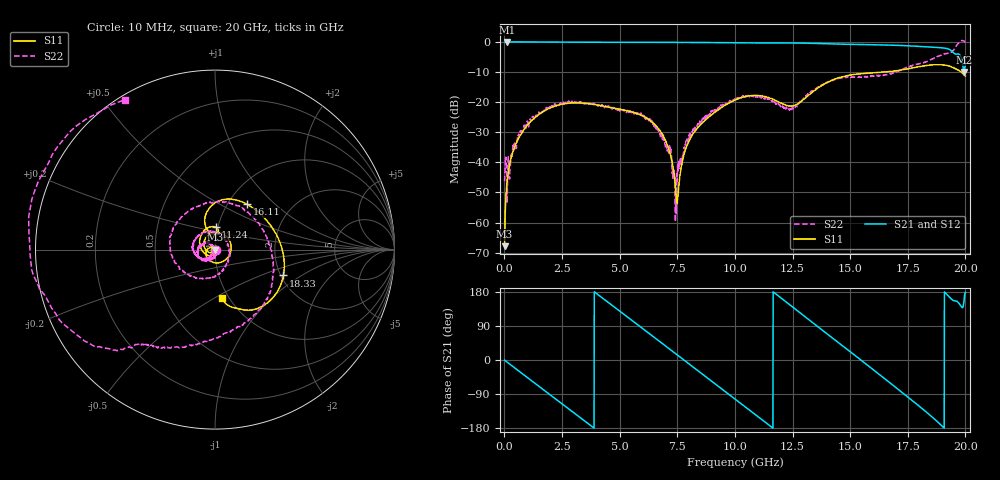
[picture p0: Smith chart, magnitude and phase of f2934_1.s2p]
!Keysight Technologies,M9372A,MY54321350,A.13.90.07
!Automatic Fixture Removal (AFR)
!Date: Wednesday, January 06, 2021, 09:20:31
!S2P File: Measurements: S11,S21,S12,S22:
# MHz S  RI  R 50
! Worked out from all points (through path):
!   2000 points, 10 MHz to 20 GHz, reference 50 ohm
!   highest |S21| = 0.03 dB at 110 MHz (marker M1); lowest = -9.9 dB at 19.94 GHz (marker M2)
!   group delay of S21, straight-line fit = 130 ps
!   lowest |S11| = -67.8 dB at 10 MHz (marker M3), VSWR 1.00, Z = 50 - j0.0401 ohm
!   |S11| at or under -10 dB: start of sweep to 16.5 GHz; 19.82 GHz to end of sweep
!   |S22| runs from -59.7 to 0.5 dB; largest |S21 - S12| = 1.4e-15
!   S11 on the Smith chart (normalised r, x): 10 MHz: 1.00, -0.00; 11.24 GHz: 0.98, +0.25; 16.11 GHz: 1.23, +0.68; 18.33 GHz: 2.07, -0.71; 20 GHz: 0.93, -0.54
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10  6.53e-05 -0.000401  1.001 -0.00816  1.001 -0.00816  0.00378 -0.00302
110  -0.00032 -0.00443  0.9996 -0.0893  0.9996 -0.0893  0.0053 0.000189
570  -0.0154 -0.0175  0.8976 -0.4467  0.8976 -0.4467  0.00109 -0.0249
1780  -0.0618 0.0397  0.1299 -0.9887  0.1299 -0.9887  -0.0467 -0.0594
3350  0.0657 0.0711  -0.8957 -0.4217  -0.8957 -0.4217  -0.1012 -0.0108
4270  0.0818 -0.0279  -0.9452 0.2919  -0.9452 0.2919  -0.0842 0.0183
5280  -0.00757 -0.0723  -0.436 0.8846  -0.436 0.8846  -0.0619 0.0304
6680  -0.0357 0.00734  0.6127 0.7702  0.6127 0.7702  -0.0207 0.0258
7500  0.00194 0.000737  0.9545 0.2282  0.9545 0.2282  -0.00469 -0.00127
8140  -0.00319 -0.0278  0.9399 -0.2749  0.9399 -0.2749  -0.0192 -0.0258
10010  -0.0801 0.0735  -0.222 -0.9425  -0.222 -0.9425  -0.1089 -0.0289
11240  0.00316 0.1255  -0.9081 -0.3201  -0.9081 -0.3201  -0.0798 0.0845
12220  0.00787 0.0885  -0.8581 0.4307  -0.8581 0.4307  0.0618 0.0509
13340  -0.0541 0.1344  -0.1658 0.9341  -0.1658 0.9341  -0.0095 -0.1539
14880  0.0313 0.275  0.8109 0.4234  0.8109 0.4234  -0.2372 0.1045
16110  0.1785 0.2521  0.7725 -0.4574  0.7725 -0.4574  0.1221 0.246
16670  0.2495 0.2015  0.4772 -0.7471  0.4772 -0.7471  0.2741 0.102
18330  0.3812 -0.1437  -0.6212 -0.5458  -0.6212 -0.5458  0.0471 -0.4688
19580  0.1361 -0.3305  -0.5721 0.2563  -0.5721 0.2563  -0.6271 -0.5466
19790  0.0787 -0.3143  -0.4707 0.3457  -0.4707 0.3457  -1.031 -0.0189
19940  0.0445 -0.2811  -0.2929 0.1247  -0.2929 0.1247  -0.7721 0.6892
20000  0.0391 -0.2688  -0.447 0.0127  -0.447 0.0127  -0.5031 0.8353
